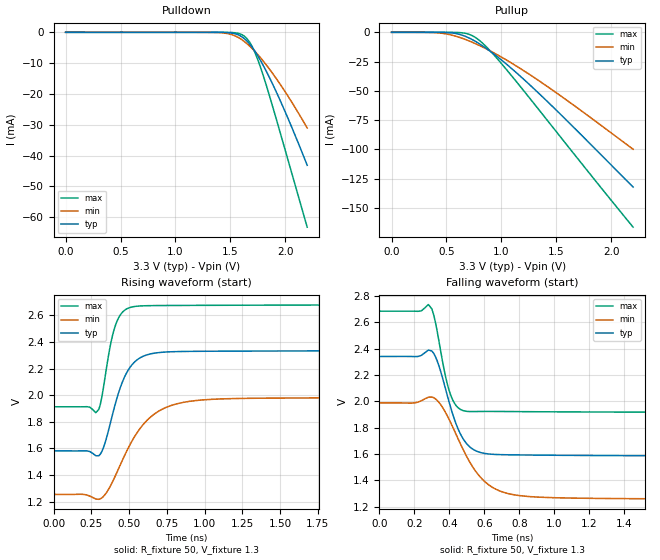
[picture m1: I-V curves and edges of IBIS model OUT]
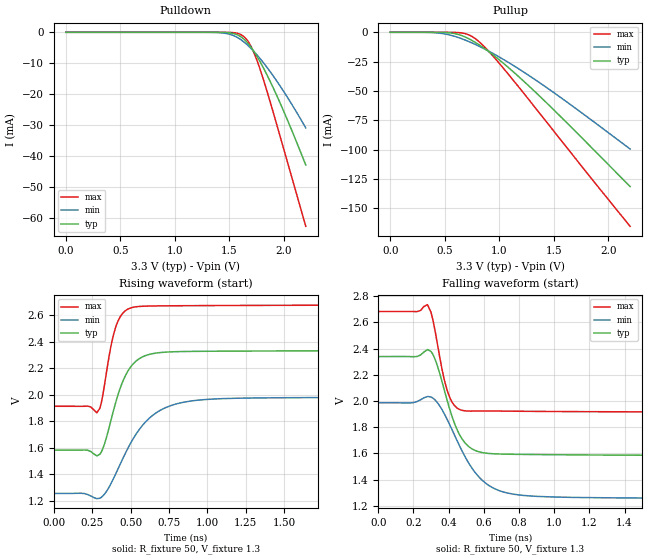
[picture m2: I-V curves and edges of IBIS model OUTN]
|   IBIS File of SG2520EHN C
|   LV-PECL, Vcc=3.3V, fo>212.5MHz
[IBIS Ver]   3.2
[File Name]   sg2520ehn_hf_33v.ibs
[File Rev]   1.0
[Date]   July 28, 2020
[Source]
[Notes]
Created by Minoru Kozaki
[Disclaimer]
Seiko Epson Corporation makes no warranty with respect to the
information contained herein.
[Copyright]
Copyright(C) 2020, Seiko Epson Corporation. All rights reserved.
|   Component
[Component]   SG2520EHN
[Manufacturer]  Seiko Epson Corporation
[Package]
R_pkg   17.7m   NA   NA
L_pkg   235p   NA   NA
C_pkg   208f   NA   NA
[Pin]   signal_name   model_name   R_pin   L_pin   C_pin
1   OE/ST   NC
2   NC   NC
3   GND   GND
4   OUT   OUT   17.7m   235p   208f
5   OUTN   OUTN   10.4m   129p   221f
6   VCC   POWER
[Diff Pin] inv_pin  vdiff  tdelay_typ
4   5   0   0
| Models and submodels in the file (2): OUT (Output_ECL), OUTN (Output_ECL)
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|   Model OUT
[Model]   OUT
Model_type   Output_ECL
Polarity   Non-Inverting
Vref = 1.3
Vmeas = 1.966
Rref = 50
Cref = 0
C_comp   0.5p   0.5p   0.5p
[Temperature Range]   25   105   -40
[Voltage Range]   3.3   2.97   3.63
[Pullup Reference]   3.3   2.97   3.63
[Pulldown Reference]   3.3   2.97   3.63
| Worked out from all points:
|   falling waveform, R_fixture 50, V_fixture 1.3: 20-80 % time 112ps typ, 187ps min, 71.6ps max; typ from 2.34 V to 1.58 V
|   rising waveform, R_fixture 50, V_fixture 1.3: 20-80 % time 130ps typ, 234ps min, 79ps max; typ from 1.58 V to 2.34 V
[Pullup]
0V        25.97nA    13.28nA    125.8nA
375mV     -8.795uA   -201.8uA   -2.71uA
550mV     -532.3uA   -2.406mA   -30.1uA
625mV     -1.893mA   -4.489mA   -259.2uA
700mV     -4.561mA   -7.115mA   -1.483mA
750mV     -6.981mA   -9.105mA   -3.574mA
800mV     -9.792mA   -11.25mA   -6.878mA
875mV     -14.56mA   -14.74mA   -13.48mA
975mV     -21.69mA   -19.8mA    -23.86mA
1.275V    -46.29mA   -37.16mA   -58.26mA
1.625V    -78.06mA   -60mA      -99.61mA
2.2V      -132.3mA   -99.96mA   -166.5mA
[Pulldown]
0V        25.97nA    13.28nA    125.8nA
1.4V      -15.89uA   -104.5uA   -3.912uA
1.475V    -101.4uA   -410.2uA   -19.3uA
1.55V     -533uA     -1.262mA   -177.8uA
1.625V    -1.974mA   -2.907mA   -1.175mA
1.675V    -3.775mA   -4.43mA    -3.139mA
1.7V      -4.922mA   -5.299mA   -4.687mA
1.75V     -7.627mA   -7.217mA   -8.855mA
1.8V      -10.76mA   -9.339mA   -14.05mA
1.875V    -16.03mA   -12.83mA   -22.82mA
1.975V    -23.8mA    -17.97mA   -35.14mA
2.2V      -43.14mA   -31.04mA   -63.21mA
[Falling Waveform]
R_fixture = 50
V_fixture = 1.3
V_fixture_min = 0.97
V_fixture_max = 1.63
0s        2.34V      1.987V     2.683V
280ps     2.388V     2.031V     2.734V
300ps     2.381V     2.032V     2.7V
330ps     2.307V     2.007V     2.533V
380ps     2.084V     1.91V      2.176V
410ps     1.941V     1.83V      2.038V
500ps     1.676V     1.578V     1.923V
640ps     1.598V     1.352V     1.923V
860ps     1.591V     1.276V     1.921V
4ns       1.582V     1.255V     1.914V
[Rising Waveform]
R_fixture = 50
V_fixture = 1.3
V_fixture_min = 0.97
V_fixture_max = 1.63
0s        1.581V     1.254V     1.913V
300ps     1.545V     1.217V     1.893V
340ps     1.637V     1.251V     2.126V
380ps     1.807V     1.325V     2.395V
410ps     1.938V     1.395V     2.526V
470ps     2.136V     1.545V     2.638V
530ps     2.242V     1.676V     2.666V
710ps     2.322V     1.889V     2.674V
1ns       2.33V      1.966V     2.676V
4ns       2.338V     1.985V     2.682V
[Ramp]
R_load = 50
dV/dt_r   0.45182/129.37p   0.43669/233.32p   0.45927/78.51p
dV/dt_f   0.45182/110.96p   0.43669/185.69p   0.45927/70.78p
|   Model OUTN
[Model]   OUTN
Model_type   Output_ECL
Polarity   Inverting
Vref = 1.3
Vmeas = 1.966
Rref = 50
Cref = 0
C_comp   0.5p   0.5p   0.5p
[Temperature Range]   25   105   -40
[Voltage Range]   3.3   2.97   3.63
[Pullup Reference]   3.3   2.97   3.63
[Pulldown Reference]   3.3   2.97   3.63
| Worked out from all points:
|   falling waveform, R_fixture 50, V_fixture 1.3: 20-80 % time 112ps typ, 188ps min, 71.6ps max; typ from 2.34 V to 1.58 V
|   rising waveform, R_fixture 50, V_fixture 1.3: 20-80 % time 131ps typ, 236ps min, 79ps max; typ from 1.58 V to 2.34 V
[Pullup]
0V        25.97nA    13.28nA    125.8nA
375mV     -8.795uA   -201.8uA   -2.71uA
550mV     -532uA     -2.403mA   -30.1uA
625mV     -1.89mA    -4.481mA   -259.1uA
700mV     -4.551mA   -7.101mA   -1.481mA
750mV     -6.962mA   -9.084mA   -3.564mA
800mV     -9.761mA   -11.23mA   -6.849mA
875mV     -14.51mA   -14.7mA    -13.41mA
975mV     -21.6mA    -19.74mA   -23.72mA
1.275V    -46.06mA   -37.02mA   -57.86mA
1.625V    -77.63mA   -59.75mA   -98.91mA
2.2V      -131.5mA   -99.49mA   -165.4mA
[Pulldown]
0V        25.97nA    13.28nA    125.8nA
1.4V      -15.89uA   -104.5uA   -3.912uA
1.475V    -101.4uA   -410uA     -19.3uA
1.55V     -532.7uA   -1.261mA   -177.7uA
1.625V    -1.971mA   -2.903mA   -1.174mA
1.675V    -3.766mA   -4.422mA   -3.13mA
1.7V      -4.91mA    -5.289mA   -4.67mA
1.75V     -7.604mA   -7.202mA   -8.81mA
1.8V      -10.72mA   -9.318mA   -13.97mA
1.875V    -15.97mA   -12.8mA    -22.67mA
1.975V    -23.69mA   -17.92mA   -34.89mA
2.2V      -42.93mA   -30.94mA   -62.76mA
[Falling Waveform]
R_fixture = 50
V_fixture = 1.3
V_fixture_min = 0.97
V_fixture_max = 1.63
0s        2.339V     1.986V     2.682V
220ps     2.339V     1.996V     2.681V
280ps     2.392V     2.034V     2.735V
300ps     2.378V     2.031V     2.677V
330ps     2.294V     1.998V     2.485V
400ps     1.967V     1.838V     2.05V
490ps     1.686V     1.584V     1.925V
630ps     1.6V       1.355V     1.924V
860ps     1.592V     1.276V     1.921V
4ns       1.582V     1.255V     1.914V
[Rising Waveform]
R_fixture = 50
V_fixture = 1.3
V_fixture_min = 0.97
V_fixture_max = 1.63
0s        1.581V     1.254V     1.913V
280ps     1.538V     1.214V     1.864V
300ps     1.55V      1.218V     1.897V
330ps     1.627V     1.248V     2.072V
370ps     1.796V     1.323V     2.354V
410ps     1.968V     1.418V     2.533V
530ps     2.248V     1.692V     2.664V
710ps     2.321V     1.892V     2.672V
1ns       2.329V     1.965V     2.674V
4ns       2.337V     1.985V     2.681V
[Ramp]
R_load = 50
dV/dt_r   0.45141/130.06p   0.43631/235.00p   0.45881/78.51p
dV/dt_f   0.45141/111.11p   0.43631/186.43p   0.45881/70.78p
